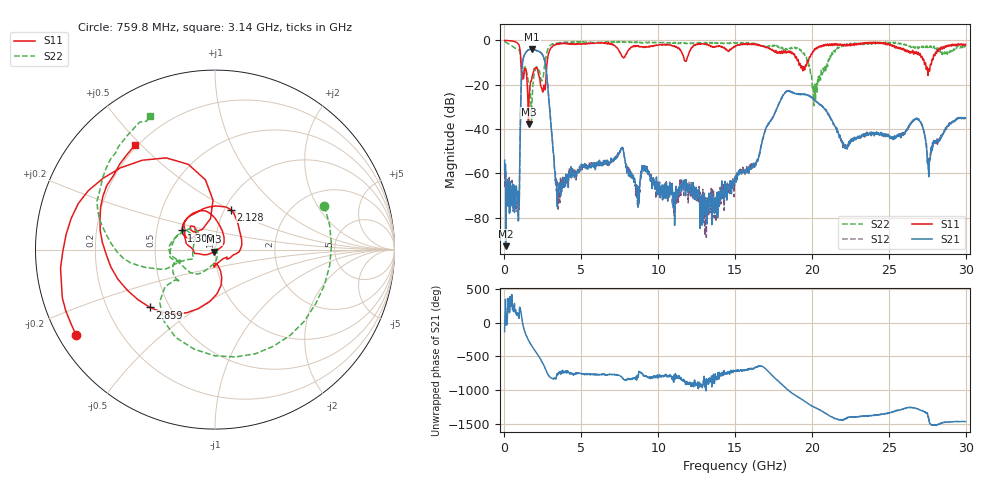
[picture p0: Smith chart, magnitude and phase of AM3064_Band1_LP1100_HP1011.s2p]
# Hz S DB R 50.0
!freq dBS11 angS11 dBS21 angS21 dBS12 angS12 dBS22 angS22
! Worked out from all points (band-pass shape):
!   1600 points, 10 MHz to 29.98 GHz, reference 50 ohm
!   highest |S21| = -3.99 dB at 1.791 GHz (marker M1); lowest = -92.9 dB at 103.7 MHz (marker M2)
!   |S21| within 3 dB of the highest: 1.273 GHz to 2.511 GHz (1.238 GHz wide, 65.4 % of centre)
!   lowest |S11| = -37.9 dB at 1.566 GHz (marker M3), VSWR 1.03, Z = 49.6 - j1.18 ohm
!   |S11| at or under -10 dB: 1.071 GHz to 2.775 GHz (1.704 GHz wide, 88.6 % of centre); 19.13 GHz to 19.68 GHz (547.1 MHz wide, 2.82 % of centre); 27.3 GHz to 27.78 GHz (478.8 MHz wide, 1.74 % of centre)
!   |S22| runs from -37.1 to -0.5 dB; largest |S21 - S12| = 0.0095
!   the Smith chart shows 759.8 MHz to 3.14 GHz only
!   S11 on the Smith chart (normalised r, x): 759.8 MHz: 0.05, -0.28; 1.303 GHz: 0.67, +0.15; 2.128 GHz: 1.07, +0.50; 2.859 GHz: 0.39, -0.33; 3.14 GHz: 0.19, +0.48
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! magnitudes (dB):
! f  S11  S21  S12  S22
! 10 MHz  0.0  -54.1  -56.3  -0.5
! 103.7 MHz  -0.1  -92.9  -64.0  -0.8
! 759.8 MHz  -0.8  -65.7  -77.1  -3.7
! 1.303 GHz  -13.4  -6.5  -6.4  -12.5
! 1.566 GHz  -37.9  -4.3  -4.3  -19.3
! 1.791 GHz  -16.7  -4.0  -4.0  -28.3
! 2.128 GHz  -12.4  -4.8  -4.6  -12.3
! 2.859 GHz  -6.3  -24.0  -24.1  -3.2
! 3.14 GHz  -2.7  -47.0  -47.0  -1.6
! 3.478 GHz  -1.8  -67.5  -71.1  -1.2
! 5.015 GHz  -1.5  -55.9  -56.6  -0.6
! 7.62 GHz  -6.9  -48.8  -48.8  -0.7
! 8.651 GHz  -2.5  -69.4  -74.1  -0.9
! 10 GHz  -2.1  -63.9  -66.0  -1.0
! 15 GHz  -2.8  -62.2  -62.9  -1.4
! 18.25 GHz  -5.0  -23.5  -23.6  -4.3
! 19.99 GHz  -6.3  -25.7  -25.8  -17.4
! 22.15 GHz  -2.5  -48.5  -48.0  -1.8
! 25 GHz  -1.5  -42.9  -43.5  -1.2
! 26.89 GHz  -5.8  -35.5  -35.7  -3.3
! 27.64 GHz  -13.8  -54.6  -55.4  -3.1
! 29.98 GHz  -1.8  -35.1  -35.2  -3.0
